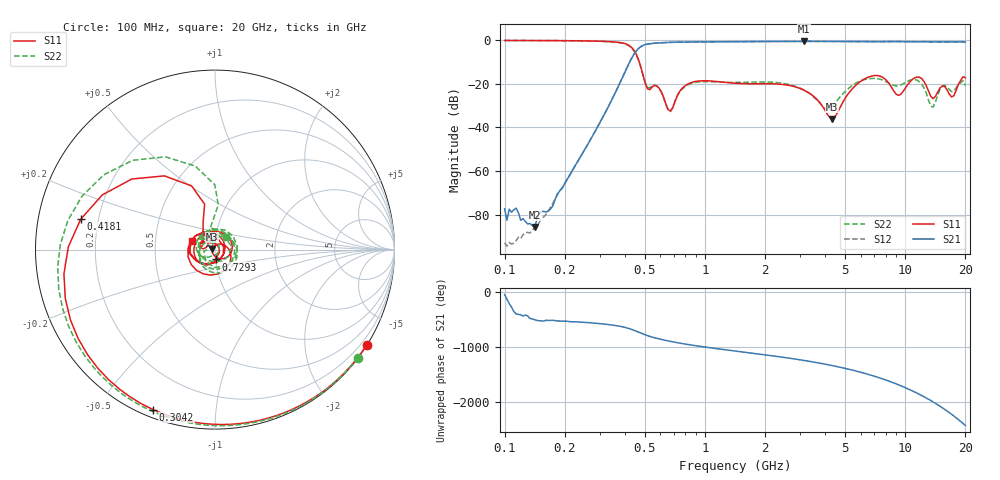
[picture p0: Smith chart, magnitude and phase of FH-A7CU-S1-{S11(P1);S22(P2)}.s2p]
!Agilent Technologies,N5230A,MY45001737,A.07.50.48
!Agilent N5230A: A.07.50.48
!Date: Wednesday, December 18, 2024 17:55:45
!Correction: S11(Full 2 Port(1,4))
!S41(Full 2 Port(1,4))
!S14(Full 2 Port(1,4))
!S44(Full 2 Port(1,4))
!S2P File: Measurements: S11, S41, S14, S44:Log Frequency Sweep
# Hz S  MA  R 50
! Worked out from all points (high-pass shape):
!   201 points, 100 MHz to 20 GHz, reference 50 ohm
!   highest |S21| = -0.44 dB at 3.131 GHz (marker M1); lowest = -85.8 dB at 141.1 MHz (marker M2)
!   |S21| within 3 dB of the highest: 470.7 MHz to end of sweep
!   lowest |S11| = -36.1 dB at 4.303 GHz (marker M3), VSWR 1.03, Z = 48.5 + j0.302 ohm
!   |S11| at or under -10 dB: 470.7 MHz to end of sweep
!   |S22| runs from -32.7 to 0.0 dB; largest |S21 - S12| = 0.023
!   S11 on the Smith chart (normalised r, x): 100 MHz: 0.01, -3.46; 304.2 MHz: 0.03, -0.68; 418.1 MHz: 0.13, +0.11; 729.3 MHz: 1.00, -0.11; 20 GHz: 0.77, +0.08
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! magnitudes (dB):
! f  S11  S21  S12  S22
! 100 MHz  0.0  -77.3  -93.0  0.0
! 141.1 MHz  0.0  -85.8  -86.1  0.0
! 169.9 MHz  -0.1  -77.4  -76.6  -0.1
! 246.1 MHz  -0.2  -51.5  -51.6  -0.2
! 304.2 MHz  -0.4  -36.5  -36.5  -0.4
! 418.1 MHz  -2.3  -10.6  -10.5  -2.5
! 516.8 MHz  -22.2  -1.7  -1.7  -21.5
! 590 MHz  -21.8  -1.2  -1.1  -22.0
! 673.6 MHz  -32.5  -0.9  -0.9  -32.7
! 729.3 MHz  -25.2  -0.8  -0.8  -25.4
! 1.414 GHz  -19.7  -0.6  -0.5  -19.3
! 3.131 GHz  -22.9  -0.4  -0.4  -22.8
! 3.481 GHz  -25.6  -0.4  -0.4  -25.8
! 4.303 GHz  -36.1  -0.5  -0.5  -30.6
! 6.072 GHz  -18.5  -0.5  -0.5  -18.4
! 8.344 GHz  -20.0  -0.6  -0.5  -19.8
! 9.276 GHz  -25.3  -0.5  -0.5  -20.8
! 11.47 GHz  -16.8  -0.6  -0.6  -18.3
! 13.8 GHz  -26.7  -0.6  -0.6  -30.7
! 15.35 GHz  -20.9  -0.7  -0.6  -21.0
! 17.06 GHz  -26.0  -0.7  -0.7  -23.5
! 20 GHz  -17.2  -0.7  -0.8  -20.8
